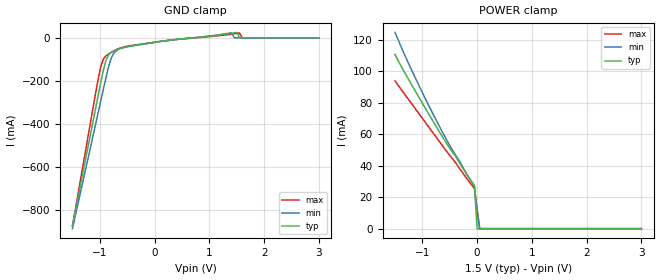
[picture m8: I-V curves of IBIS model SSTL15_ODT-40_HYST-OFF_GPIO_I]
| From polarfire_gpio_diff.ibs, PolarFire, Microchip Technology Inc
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|   Model SSTL15_ODT-40_HYST-OFF_GPIO_I
[Model]   SSTL15_ODT-40_HYST-OFF_GPIO_I
Model_type   Input
Vinl =   0.65
Vinh =   0.85
|   typ   min   max
C_comp_pullup   2.605e-12   2.605e-12   2.76e-12
C_comp_pulldown  2.605e-12   2.605e-12   2.76e-12
[Temperature Range]  25C   100C   -40C
[Voltage Range]  1.5   1.425   1.575
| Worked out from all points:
|   POWER clamp passes 1 mA (typ) near -0.00 V on its own axis
[GND Clamp]
| Voltage   I(typ)   I(min)   I(max)
-1.5V     -875.5mA   -888.5mA   -876mA
-1.034V   -271.9mA   -351.8mA   -195.6mA
-984.4mV  -209.1mA   -295.1mA   -134.7mA
-885.9mV  -103.8mA   -182.5mA   -83.59mA
-787.5mV  -66.79mA   -91.63mA   -66.89mA
-738.3mV  -60.07mA   -68.76mA   -59.92mA
-443mV    -38.5mA    -39.39mA   -36.7mA
1.406V    21.1mA     23.72mA    17mA
1.453V    23.07mA    0A         18.69mA
1.549V    0A         0A         22.44mA
1.598V    0A         0A         0A
3V        0A         0A         0A
[POWER Clamp]
| Voltage   I(typ)   I(min)   I(max)
-1.5V     110.7mA    124.8mA    93.96mA
-1.23V    93.61mA    103.4mA    81.08mA
-984.4mV  78.81mA    85.39mA    69.41mA
-787.5mV  67.25mA    71.66mA    60.06mA
-492.2mV  50.61mA    52.4mA     46.25mA
-393.7mV  46.05mA    46.82mA    41.92mA
-196.9mV  34.85mA    35.24mA    32.29mA
-49.22mV  27.41mA    27.07mA    25.62mA
0V        0A         10.4mA     12.84mA
46.88mV   0A         0A         0A
3V        0A         0A         0A
